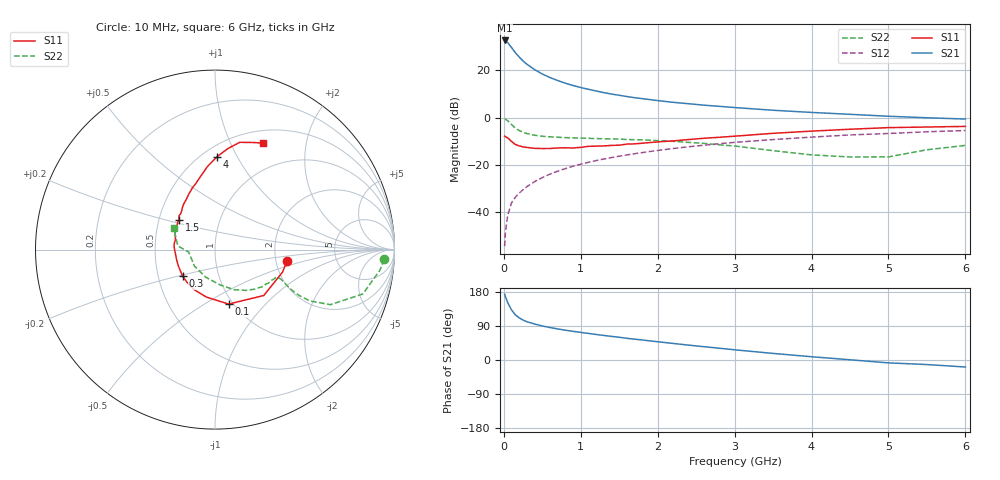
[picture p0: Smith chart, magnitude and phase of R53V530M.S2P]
! SIEMENS Small Signal Semiconductors
! BFR183
! Si NPN RF Bipolar Junction Transistor in SOT23
! VCE = 3.5 V  IC = 30 mA
! Common Emitter S-Parameters:  May  1996
# GHz  S  MA  R  50
!  f  S11  S21  S12  S22
! GHz  MAG  ANG  MAG  ANG  MAG  ANG  MAG  ANG
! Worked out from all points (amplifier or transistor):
!   36 points, 10 MHz to 6 GHz, reference 50 ohm
!   highest |S21| = 32.7 dB at 10 MHz (marker M1)
!   |S21| within 3 dB of that: start of sweep to 99.92 MHz
!   unconditionally stable (mu >= 1): 431.4 MHz to 2.329 GHz
!   at 250 MHz: K = 0.89, MSG = 27.2 dB, |S12| = -30.5 dB
!   at 1.4 GHz: K = 1.05, MAG = 12.1 dB, |S12| = -16.9 dB
!   at 6 GHz: K = 0.90, MSG = 2.4 dB, |S12| = -5.5 dB
!   S11 on the Smith chart (normalised r, x): 10 MHz: 2.30, -0.36; 100 MHz: 0.95, -0.64; 300 MHz: 0.67, -0.21; 1.5 GHz: 0.63, +0.23; 4 GHz: 0.59, +0.83; 6 GHz: 0.65, +1.33
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0.01  0.4058 -9.3  42.95 173.7  0.0019 91.7  0.9441 -3.3
0.02  0.3967 -18.5  42.35 167.5  0.0036 82.4  0.9264 -7.1
0.05  0.3729 -43.3  38.74 151.6  0.0086 75.9  0.8598 -16.7
0.1  0.3128 -76.0  30.4 132.1  0.0156 71.9  0.7126 -25.5
0.15  0.2687 -100.5  23.67 119.1  0.0207 69.9  0.6021 -28.4
0.2  0.2517 -117.1  19.11 111.2  0.0253 71.5  0.5329 -28.6
0.25  0.2399 -130.3  15.79 105.4  0.0298 71.7  0.4885 -27.9
0.3  0.2336 -140.3  13.47 101.0  0.0346 73.1  0.4598 -27.0
0.4  0.2237 -155.3  10.37 95.0  0.0441 73.6  0.4233 -25.3
0.5  0.2215 -165.8  8.369 89.8  0.0535 74.0  0.403 -24.2
0.6  0.2218 -174.8  7.044 85.7  0.0637 73.9  0.392 -23.9
0.8  0.2297 171.8  5.343 78.6  0.0833 73.1  0.3772 -24.4
0.9  0.2273 165.9  4.781 75.6  0.0937 72.3  0.372 -24.9
1.1  0.2463 155.6  3.969 70.2  0.1133 70.9  0.3646 -27.2
1.3  0.2518 147.3  3.378 64.8  0.1329 68.8  0.3569 -29.3
1.5  0.261 140.4  2.97 60.0  0.1523 66.8  0.3505 -32.3
2.2  0.3213 120.1  2.106 43.7  0.2215 59.2  0.3147 -44.4
3.5  0.4649 95.2  1.431 17.4  0.3431 42.3  0.1997 -81.4
4  0.5178 88.7  1.287 8.6  0.3861 36.2  0.1624 -108.2
4.5  0.5671 82.8  1.174 0.6  0.4298 29.4  0.1468 -141.1
5.5  0.6322 70.7  0.992 -12.0  0.5007 17.6  0.2085 174.3
6  0.6505 65.9  0.932 -18.5  0.5336 10.0  0.2579 152.8
